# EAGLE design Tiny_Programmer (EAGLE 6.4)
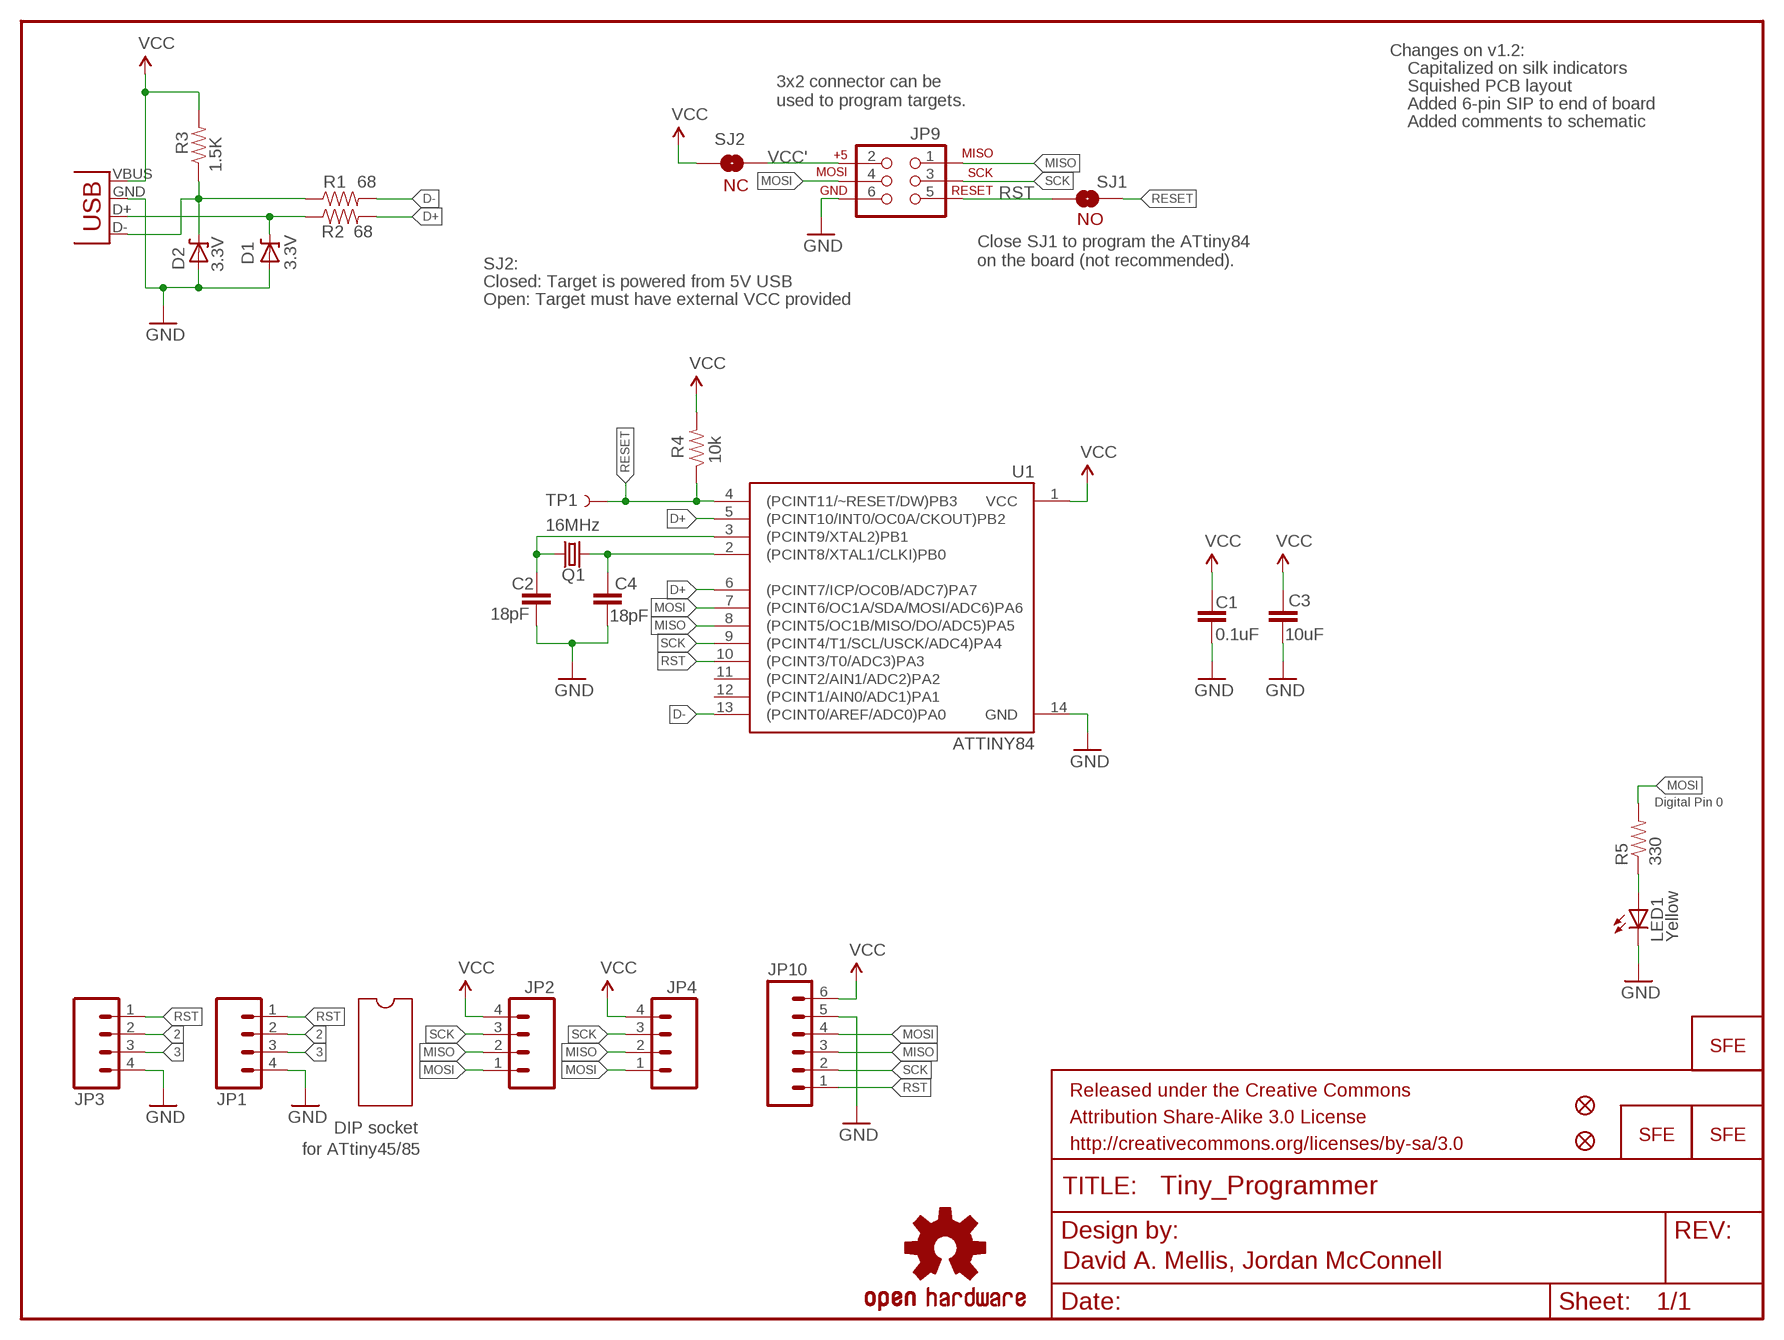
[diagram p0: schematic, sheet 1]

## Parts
C1  0.1uF  CAP0402-CAP  [0402-CAP]
C2  18pF  CAP0402-CAP  [0402-CAP]
C3  10uF  CAP0402-CAP  [0402-CAP]
C4  18pF  CAP0402-CAP  [0402-CAP]
D1  3.3V  DIODE-ZENER-BZT52  [SOD-323]
D2  3.3V  DIODE-ZENER-BZT52  [SOD-323]
FRAME1  FRAME-LETTER  [CREATIVE_COMMONS]
JP1  M04PTH  [1X04]
JP2  M04PTH  [1X04]
JP3  M04SMD_STRAIGHT_COMBO  [1X04_SMD_STRAIGHT_COMBO]
JP4  M04SMD_STRAIGHT_COMBO  [1X04_SMD_STRAIGHT_COMBO]
JP5  LOGO-SFENW2  [SFE-NEW-WEB]
JP6  LOGO-SFESK  [SFE-LOGO-FLAME]
JP7  FIDUCIALUFIDUCIAL  [MICRO-FIDUCIAL]
JP8  FIDUCIALUFIDUCIAL  [MICRO-FIDUCIAL]
JP9  AVR_SPI_PRG_6PTH  [2X3]
JP10  M06SIP  [1X06]
JP11  LOGO-SFESK  [SFE-LOGO-FLAME]
LED1  Yellow  LED0603  [LED-0603]
Q1  16MHz  CRYSTAL5X3  [CRYSTAL-SMD-5X3]
R1  68  RESISTOR0402-RES  [0402-RES]
R2  68  RESISTOR0402-RES  [0402-RES]
R3  1.5K  RESISTOR0402-RES  [0402-RES]
R4  10k  RESISTOR0402-RES  [0402-RES]
R5  330  RESISTOR0402-RES  [0402-RES]
SJ1  SOLDERJUMPERNO  [SJ_2S-NO]
SJ2  NC  SOLDERJUMPERNC  [SJ_2S]
TP1  TEST-POINT3  [PAD.03X.03]
U1  ATTINY84  [SO14]
U$1  OSHW-LOGOS  [OSHW-LOGO-S]
X1  USB-A-H  [USB-A-H]

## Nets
2: JP1.2 JP3.2
3: JP1.3 JP3.3
D+: R2.2 U1.5((PCINT10/INT0/OC0A/CKOUT)PB2) U1.6((PCINT7/ICP/OC0B/ADC7)PA7)
D-: R1.2 U1.13((PCINT0/AREF/ADC0)PA0)
GND: C1.2 C2.2 C3.2 C4.2 D1.2(A) D2.2(A) JP1.4 JP3.4 JP9.6 JP10.5 LED1.C U1.14(GND) X1.GND(VBUS)
MISO: JP2.2 JP4.2 JP9.1 JP10.3 U1.8((PCINT5/OC1B/MISO/DO/ADC5)PA5)
MOSI: JP2.1 JP4.1 JP9.4 JP10.4 R5.2 U1.7((PCINT6/OC1A/SDA/MOSI/ADC6)PA6)
N$1: D2.1(C) R1.1 R3.1 X1.D-(D+)
N$2: D1.1(C) R2.1 X1.D+(D-)
N$3: C2.1 Q1.3 U1.3((PCINT9/XTAL2)PB1)
N$4: C4.1 Q1.1 U1.2((PCINT8/XTAL1/CLKI)PB0)
N$5: LED1.A R5.1
RESET: R4.1 SJ1.1 TP1.P$1 U1.4((PCINT11/~RESET/DW)PB3)
RST: JP1.1 JP3.1 JP9.5 JP10.1 SJ1.2 U1.10((PCINT3/T0/ADC3)PA3)
SCK: JP2.3 JP4.3 JP9.3 JP10.2 U1.9((PCINT4/T1/SCL/USCK/ADC4)PA4)
VCC: C1.1 C3.1 JP2.4 JP4.4 JP10.6 R3.2 R4.2 SJ2.1 U1.1(VCC) X1.VBUS(GND)
VCC': JP9.2 SJ2.2
Unconnected: U1.11((PCINT2/AIN1/ADC2)PA2) U1.12((PCINT1/AIN0/ADC1)PA1)

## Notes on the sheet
- Changes on v1.2:
- Capitalized on silk indicators
- Squished PCB layout
- 3x2 connector can be
  used to program targets.
- Added 6-pin SIP to end of board
- Added comments to schematic
- NC
- NO
- Close SJ1 to program the ATtiny84
  on the board (not recommended).
- SJ2:
- Closed: Target is powered from 5V USB
- Open: Target must have external VCC provided
- Digital Pin 0
- DIP socket
- for ATtiny45/85
- David A. Mellis, Jordan McConnell

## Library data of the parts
C1-C4 = SparkFun-Passives:CAP: Capacitor
D1 D2 = SparkFun-DiscreteSemi:DIODE-ZENER: Zener Diode
FRAME1 = SparkFun-Aesthetics:FRAME-LETTER: Schematic Frame
JP1-JP4 = SparkFun-Connectors:M04: Header 4 Standard 4-pin 0.1" header. Use with straight break away headers (SKU : PRT-00116), right angle break away headers (PRT-00553), swiss pins (PRT-00743), machine pins (PRT-00117), and female headers (PRT-00115). Molex polarized connector foot print use with SKU : PRT-08231 with associated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
JP5 JP6 JP11 = SparkFun-Aesthetics:LOGO-SFE: Spark Fun Electronics PCB Logo
JP7 JP8 = SparkFun:FIDUCIAL: Fiducial Alignment Points
JP9 = SparkFun-Connectors:AVR_SPI_PRG_6: AVR ISP 6 Pin This is the reduced ISP connector for AVR programming. Common on Arduino. This footprint will take up less PCB space and can be used with a 10-pin to 6-pin adapter such as SKU: BOB-08508
JP10 = SparkFun-Connectors:M06: Header 6 Standard 6-pin 0.1" header. Use with straight break away headers (SKU : PRT-00116), right angle break away headers (PRT-00553), swiss pins (PRT-00743), machine pins (PRT-00117), and female headers (PRT-00115). Molex polarized connector foot print use with SKU : PRT-08094 with associated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
LED1 = SparkFun-LED:LED: LEDs
Q1 = SparkFun-FreqCtrl:CRYSTAL: Various standard crystals. Proven footprints. Spark Fun Electronics SKU : COM-00534
R1-R5 = SparkFun-Passives:RESISTOR: Resistor
SJ1 SJ2 = SparkFun-Passives:SOLDERJUMPER: Solder Jumper
TP1 = SparkFun-Passives:TEST-POINT: Bare copper test points for troubleshooting or ICT
U1 = SparkFun-DigitalIC:ATTINY84: Atmel 14-pin 2/4/8kB flash uC
U$1 = SparkFun-Aesthetics:OSHW-LOGO: Open Source Hardware Logo This logo indicates the piece of hardware it is found on incorporates a OSHW license and/or adheres to the definition of open source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
X1 = SparkFun-Connectors:USB: USB Connectors USB-B-PTH is fully proven SKU : PRT-00139 USB-miniB is fully proven SKU : PRT-00587 USB-A-PCB is untested. USB-A-H is throughly reviewed, but untested. Spark Fun Electronics SKU : PRT-00437 USB-B-SMT is throughly reviewed, but untested. Needs silkscreen touching up. USB-A-S has not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

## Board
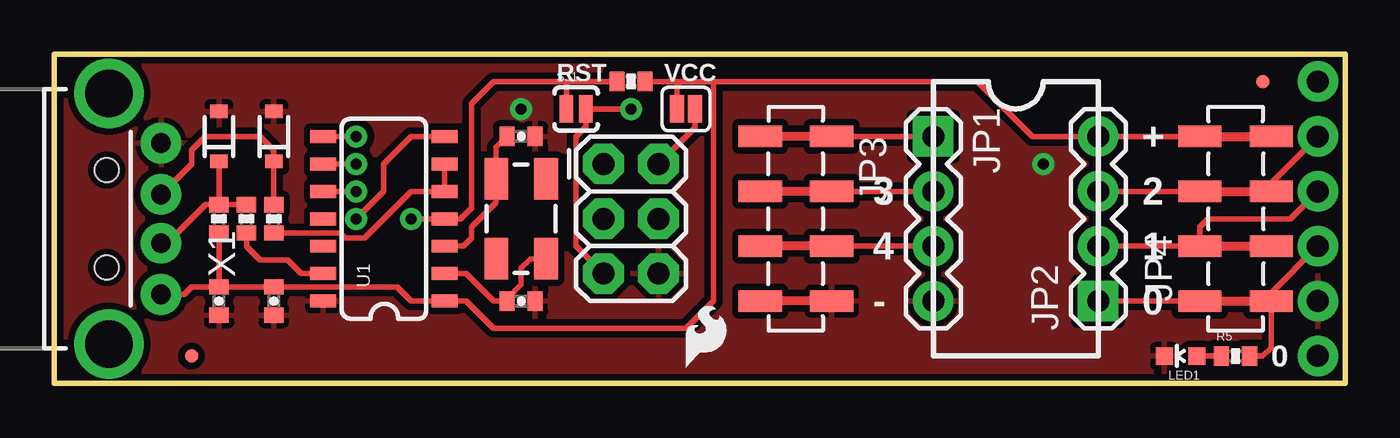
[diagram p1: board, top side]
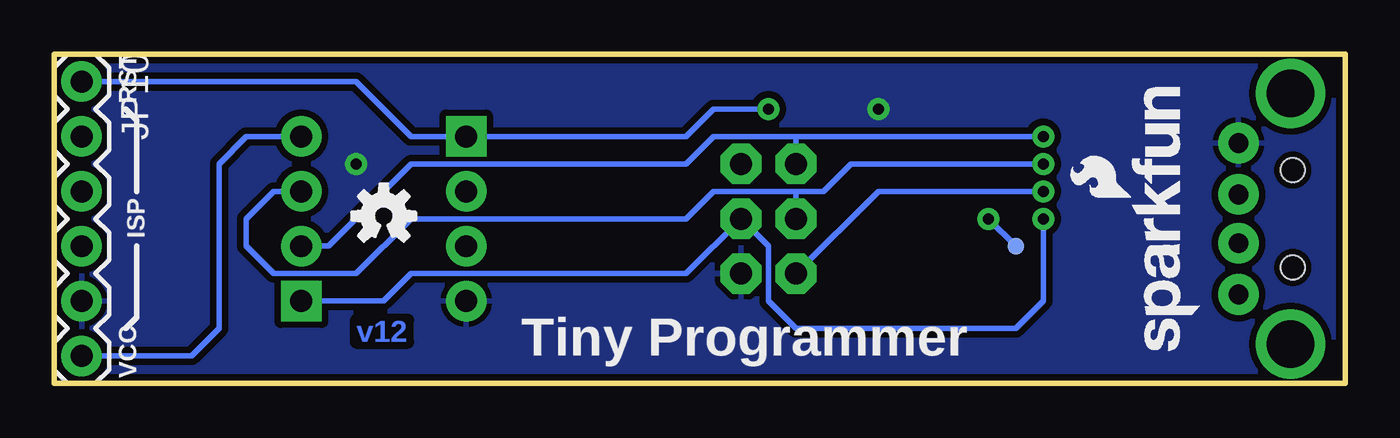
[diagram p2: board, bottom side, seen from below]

Size 59.69 x 15.24 mm. Coordinates in mm from the lower left corner, seen from the top.
Outline: 0,0 59.69,0 59.69,15.24 0,15.24 0,0
Copper layers (1*16): Top 0.035mm / dielectric 1.5mm / Bottom 0.035mm
Design rules "default": minimum track width 8mil, minimum drill 20mil, track to track 8mil, track to pad 8mil, pad to pad 8mil, via to via 8mil, smd to smd 8mil, copper to edge 8mil, drill to drill 8mil, minimum pad ring 12mil, minimum via ring 10mil, stop-mask expansion 4mil, vias tented up to drill 20mil, thermal gap 10mil

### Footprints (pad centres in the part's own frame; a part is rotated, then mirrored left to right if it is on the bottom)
0402-CAP = smd 0.7 x 0.9: 1 -0.65,0; 2 0.65,0
SOD-323 = smd 0.63 x 0.83: 1 -1.15,0; 2 1.15,0
1X04 = drill 1.016 pad 1.88 square: 1 0,0 | drill 1.016 pad 1.88: 2 2.54,0; 3 5.08,0; 4 7.62,0
1X04_SMD_STRAIGHT_COMBO = smd 1 x 2: 1 0,-1.65; 1-2 0,1.65; 2 2.54,1.65; 2-2 2.54,-1.65; 3 5.08,-1.65; 3-2 5.08,1.65; 4 7.62,1.65; 4-2 7.62,-1.65
MICRO-FIDUCIAL = smd 0.635 x 0.635: 1 0,0
2X3 = drill 1.016 pad 1.88 octagon: 1 0,0; 2 0,2.54; 3 2.54,0; 4 2.54,2.54; 5 5.08,0; 6 5.08,2.54
1X06 = drill 1.016 pad 1.88: 1 0,0; 2 2.54,0; 3 5.08,0; 4 7.62,0; 5 10.16,0; 6 12.7,0
LED-0603 = smd 0.8 x 0.8: A 0,-0.75; C 0,0.75
CRYSTAL-SMD-5X3 = smd 1.9 x 1.1: 1 -1.85,-1.15; 2 1.85,-1.15; 3 1.85,1.15; 4 -1.85,1.15
0402-RES = smd 0.7 x 0.9: 1 -0.65,0; 2 0.65,0
SJ_2S-NO = smd 0.635 x 1.27: 1 -0.45,0; 2 0.45,0
SJ_2S = smd 0.635 x 1.27: 1 -0.412,0; 2 0.412,0
PAD.03X.03 = smd 0.762 x 0.762: P$1 0,0
SO14 = smd 0.6 x 1.2: 1 -3.81,-2.8; 2 -2.54,-2.8; 3 -1.27,-2.8; 4 0,-2.8; 5 1.27,-2.8; 6 2.54,-2.8; 7 3.81,-2.8; 8 3.81,2.8; 9 2.54,2.8; 10 1.27,2.8; 11 0,2.8; 12 -1.27,2.8; 13 -2.54,2.8; 14 -3.81,2.8
USB-A-H = drill 0.914 pad 1.88: D+ 2.4,1.127; D- 2.4,-1.127; GND 2.4,3.5; VBUS 2.4,-3.5 | drill 2.2: GND2 0,-5.8; GND3 0,5.8 | hole 1.1: -0.1,2.25; -0.1,-2.25

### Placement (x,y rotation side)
C1  7.62,3.81 270 top
C2  21.59,11.43 0 top
C3  10.16,3.81 270 top
C4  21.59,3.81 0 top
D1  10.16,11.43 90 top
D2  7.62,11.43 90 top
FRAME1  not placed on the board
JP1  40.64,11.43 270 top
JP2  48.26,3.81 90 top
JP3  34.29,11.43 270 top
JP4  54.61,3.81 90 top
JP5  6.73,1.52 90 bottom
JP6  29.21,0.76 0 top
JP7  6.35,1.27 0 top
JP8  55.88,13.97 0 top
JP9  25.4,10.16 270 top
JP10  58.42,13.97 270 bottom
JP11  9.91,8.64 90 bottom
LED1  52.07,1.27 90 top
Q1  21.59,7.62 90 top
R1  8.89,7.62 270 top
R2  10.16,7.62 270 top
R3  7.62,7.62 270 top
R4  26.67,13.97 0 top
R5  54.61,1.27 0 top
SJ1  24.13,12.7 0 top
SJ2  29.21,12.7 0 top
TP1  15.24,6.35 0 bottom
U1  15.24,7.62 90 top
U$1  44.45,7.75 0 bottom
X1  2.54,7.62 0 top

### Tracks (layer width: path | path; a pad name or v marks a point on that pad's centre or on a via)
2
  Top 0.254: JP1.2 JP3.2
3
  Top 0.254: JP1.3 JP3.3
D+
  Top 0.254: U1.6 U1.5 16.51,8.89 14.35,6.73 13.46,6.73 13.22,6.97 R2.2
D-
  Top 0.254: R1.2 8.9,6.97 8.9,6.33 9.53,5.71 10.79,5.71 11.43,5.08 U1.13
GND  (via drill 0.51)
  other vias: 45.72,10.16 21.59,12.7
  pour Bottom (isolate 0.305): 0,0 0,15.24 59.69,15.24 59.69,0
  pour Top (isolate 0.305): 0,0 0,15.24 59.69,15.24 59.69,0
MISO  (via drill 0.51)
  Top 0.254: JP2.2 JP4.2 52.96,7.24 53.34,7.62 57.15,7.62 JP10.3 | U1.8 v13.97,11.43
  Bottom 0.254: v13.97,11.43 25.4,11.43 | 25.4,11.43 29.21,11.43 30.48,10.16 43.18,10.16 46.99,6.35 JP2.2 | JP9.1 25.4,11.43
MOSI  (via drill 0.51)
  Top 0.254: JP2.1 JP4.1 | R5.2 55.88,1.27 56.26,1.65 JP4.1 | U1.7 16.51,11.43 15.24,10.16 15.24,8.89 v13.97,7.62 | JP4.1 56.26,4.19 JP10.4
  Bottom 0.254: v13.97,7.62 13.97,3.81 15.24,2.54 25.4,2.54 26.67,3.81 26.67,6.35 JP9.4 30.48,5.08 43.18,5.08 44.45,3.81 JP2.1
N$1
  Top 0.254: R3.1 R1.1 | D2.1 R3.1 | R3.1 7,8.27 5.22,6.49 X1.D-
N$2
  Top 0.254: X1.D+ 6.35,10.16 6.35,10.79 6.99,11.43 9.53,11.43 10.16,10.79 D1.1 R2.1
N$3
  Top 0.254: U1.3 18.92,6.35 19.3,6.73 19.3,7.24 20.44,8.38 Q1.3 20.44,10.93 C2.1
N$4
  Top 0.254: U1.2 19.05,5.08 20.32,3.81 C4.1 20.94,3.92 21.59,4.57 21.59,5.33 22.03,5.77 Q1.1
N$5
  Top 0.254: R5.1 LED1.A
RESET  (via drill 0.51)
  Top 0.254: v16.51,7.62 U1.4 18.8,7.62 19.3,8.13 19.3,12.95 20.32,13.97 23.62,13.97 | SJ1.1 23.68,13.91 23.62,13.97 | 23.62,13.97 R4.1
  Bottom 0.254: v16.51,7.62 TP1.P$1
RST  (via drill 0.51)
  Top 0.254: U1.10 v13.97,8.89 | JP3.1 JP1.1 | JP9.5 24.13,6.35 24.13,11.43 24.58,11.88 SJ1.2 v26.67,12.7
  Bottom 0.254: v13.97,8.89 21.59,8.89 JP9.5 | v26.67,12.7 29.21,12.7 30.48,11.43 JP1.1 43.18,11.43 45.72,13.97 JP10.1
SCK  (via drill 0.51)
  Top 0.254: v13.97,10.16 U1.9 | JP10.2 56.26,9.27 JP4.3 JP2.3
  Bottom 0.254: v13.97,10.16 22.86,10.16 24.13,8.89 25.4,8.89 | 25.4,8.89 29.21,8.89 30.48,7.62 43.18,7.62 45.72,5.08 49.53,5.08 50.8,6.35 50.8,7.62 49.53,8.89 JP2.3 | JP9.3 25.4,8.89
VCC
  Top 0.254: JP4.4 JP2.4 45.21,11.43 42.67,13.97 30.48,13.97 | R3.2 C1.1 | C1.1 C3.1 15.86,4.46 16.51,3.81 U1.1 19.05,3.81 20.32,2.54 29.21,2.54 30.48,3.81 30.48,13.97 | SJ2.1 28.8,13.81 28.96,13.97 | R4.2 28.96,13.97 | 28.96,13.97 30.48,13.97 | X1.VBUS 6.03,4.12 6.37,4.46 C1.1
  Bottom 0.254: JP10.6 53.34,1.27 52.07,2.54 52.07,10.16 50.8,11.43 JP2.4
VCC'
  Top 0.254: SJ2.2 29.62,11.84 JP9.2

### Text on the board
Bottom: v12
tPlace: RST | VCC | + | 3 | 2 | 4 | 1 | - | 0 | 0
bPlace: RST | ISP | Tiny Programmer | VCC
tNames: MIT Media Lab | High-Low Tech | hlt.media.mit.edu
tValues: David A. Mellis, Jordan McConnell

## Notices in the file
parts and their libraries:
SparkFun-Passives: Licensing: CC v3.0 Share-Alike You are welcome to use this library for commercial purposes.
SparkFun-Aesthetics: Released under the Creative Commons Attribution Share-Alike 3.0 License
SparkFun-Aesthetics: http://creativecommons.org/licenses/by-sa/3.0
